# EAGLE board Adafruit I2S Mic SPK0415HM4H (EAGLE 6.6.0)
REV: A
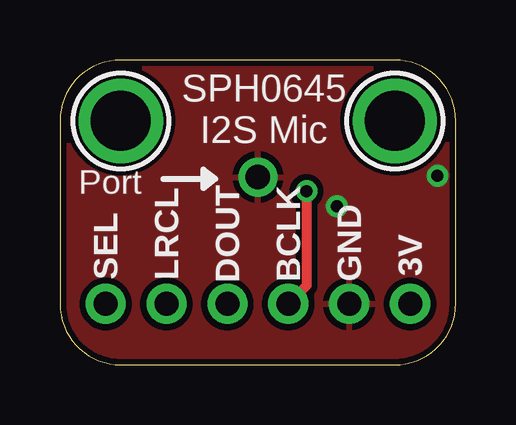
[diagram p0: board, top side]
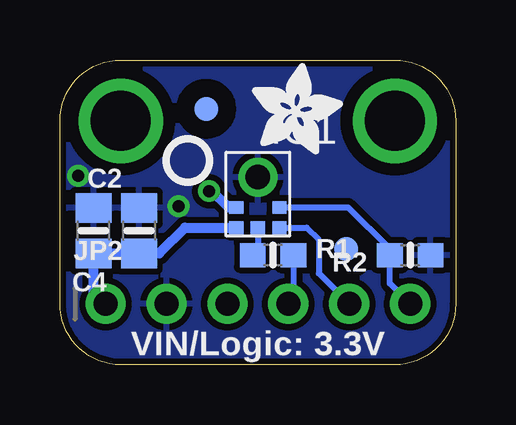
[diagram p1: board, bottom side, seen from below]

Size 16.51 x 12.7 mm. Coordinates in mm from the lower left corner, seen from the top.
Outline: 0,10.16 0,2.54 arc90 2.54,0 13.97,0 arc90 16.51,2.54 16.51,10.16 arc90 13.97,12.7 2.54,12.7 arc90 0,10.16
Copper layers (1*16): Top 0.035mm / dielectric 1.5mm / Bottom 0.035mm
Design rules "adafruit": minimum track width 8mil, minimum drill 15.5mil, track to track 8mil, track to pad 8mil, pad to pad 8mil, via to via 8mil, smd to smd 8mil, copper to edge 10mil, drill to drill 8mil, minimum pad ring 10mil, minimum via ring 8mil, stop-mask expansion 2mil, vias tented up to drill 20mil, thermal gap 10mil

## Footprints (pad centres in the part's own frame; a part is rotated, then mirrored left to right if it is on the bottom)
0805-NO = smd 1.24 x 1.5: 1 -0.95,0; 2 0.95,0
FIDUCIAL_1MM = smd 1 x 1: 1 0,0
SPH0645LM4H = smd 0.6 x 0.525: 1 -0.9,1.4; 2 -0.9,0.55; 4 0.9,0.55; 5 0.9,1.4; 6 0,1.4 | drill 1.025 pad 1.625: 3 0,-0.71
1X06_ROUND = drill 1 pad 1.676: 1 -6.35,0; 2 -3.81,0; 3 -1.27,0; 4 1.27,0; 5 3.81,0; 6 6.35,0
0603-NO = smd 1.075 x 1: 1 -0.85,0; 2 0.85,0
MOUNTINGHOLE_2.5_PLATED = drill 2.5 pad 3.2: P$1 0,0

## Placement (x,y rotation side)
C2  220pF  [0805-NO]  13.21,5.59 90 bottom
C4  1uF  [0805-NO]  15.11,5.59 90 bottom
FID1  FIDUCIAL_1MM  [FIDUCIAL_1MM]  10.41,10.67 0 bottom
FID2  FIDUCIAL_1MM  [FIDUCIAL_1MM]  4.57,4.83 0 bottom
IC1  MIC_I2S_SPH0645  [SPH0645LM4H]  8.26,7.11 180 bottom
JP2  [1X06_ROUND]  8.26,2.54 0 bottom
R1  68  [0603-NO]  7.62,4.57 0 bottom
R2  10k  [0603-NO]  1.9,4.57 180 bottom
U$5  [ADAFRUIT_3.5MM]  8.51,8.76 0 bottom
U$6  MOUNTINGHOLE2.5  [MOUNTINGHOLE_2.5_PLATED]  2.54,10.16 0 top
U$12  MOUNTINGHOLE2.5  [MOUNTINGHOLE_2.5_PLATED]  13.97,10.16 0 top
U$13  [PCBFEAT-REV-040]  11.18,8.51 0 bottom

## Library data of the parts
C2 C4 IC1 JP2 R1 R2 U$5 U$13 = microbuilder
FID1 FID2 U$6 U$12 = microbuilder; BOM: EXCLUDE

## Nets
BCLK: IC1.4 JP2.3
DATA: JP2.4 R1.2
GND: C2.2 C4.2 IC1.3 JP2.2 R2.1
N$1: IC1.6 R1.1
SELECT: IC1.2 JP2.6 R2.2
VDD: C2.1 C4.1 IC1.5 JP2.1
WS: IC1.1 JP2.5

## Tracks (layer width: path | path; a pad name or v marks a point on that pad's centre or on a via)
BCLK  (via drill 0.5)
  Top 0.406: v10.29,7.24 10.29,3.3 JP2.3
  Bottom 0.406: IC1.4 9.48,6.56 10.16,7.24 v10.29,7.24
DATA
  Bottom 0.254: R1.2 6.77,2.75 JP2.4
GND  (via drill 0.5)
  other vias: 15.75,7.87 11.56,6.6
  pour Bottom (isolate 0.254): 0,0 16.51,0 16.51,12.7 0,12.7
  pour Top (isolate 0.254): 0,0 16.51,0 16.51,12.7 0,12.7
N$1
  Bottom 0.254: IC1.6 8.26,4.45 R1.1
SELECT
  Bottom 0.254: IC1.2 4.49,6.56 2.75,4.83 R2.2 2.75,3.39 JP2.6
VDD
  Bottom 0.406: JP2.1 15.11,3.05 C4.1 C2.1 | C2.1 12.63,4.64 | IC1.5 11.3,5.71 12.37,4.64 C2.1
WS
  Bottom 0.254: IC1.1 6.22,5.71 5.71,5.21 5.71,3.81 JP2.5

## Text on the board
tPlace: SPH0645 / I2S Mic | Port | SEL | LRCL | DOUT | BCLK | GND | 3V
bPlace: VIN/Logic: 3.3V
